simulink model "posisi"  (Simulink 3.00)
settings: Solver=ode45  StartTime=0.0  StopTime=20  RelTol=1e-3

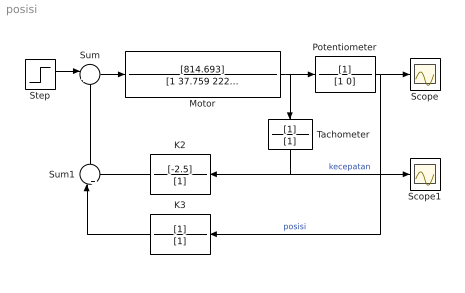
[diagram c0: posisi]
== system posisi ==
  K2 : TransferFcn  Orientation=left  Numerator=[-2.5]  Denominator=[1]
  K3 : TransferFcn  Orientation=left  Numerator=[1]  Denominator=[1]
  Motor : TransferFcn  Numerator=[814.693]  Denominator=[1 37.759 2222.617]
  Potentiometer : TransferFcn  Numerator=[1]  Denominator=[1 0]
  Scope : Scope
  Scope1 : Scope
  Step : Step  Time=0  Before=0  After=1  SampleTime=0.01
  Sum : Sum  Inputs=|+-  SaturateOnIntegerOverflow=on
  Sum1 : Sum  Orientation=up  Inputs=|++  SaturateOnIntegerOverflow=on
  Tachometer : TransferFcn  Orientation=down  Numerator=[1]  Denominator=[1]
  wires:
  Sum/1 -> Motor/1
  Step/1 -> Sum/1
  Potentiometer/1 -> Scope/1, K3/1  "posisi"
  Motor/1 -> Potentiometer/1, Tachometer/1
  Sum1/1 -> Sum/2
  K3/1 -> Sum1/1
  K2/1 -> Sum1/2
  Tachometer/1 -> K2/1, Scope1/1  "kecepatan"
